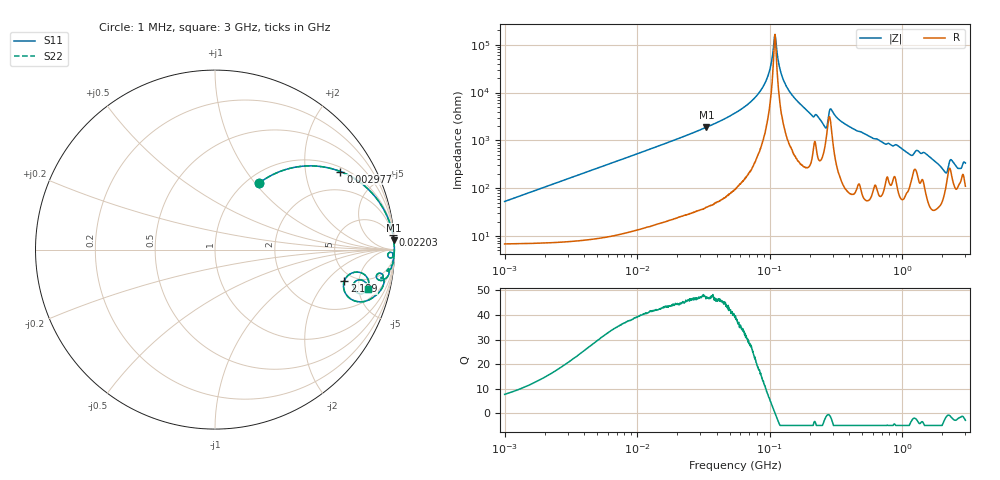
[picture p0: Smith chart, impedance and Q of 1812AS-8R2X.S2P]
!s-Parameter Generated by FASTRON Sdn. Bhd.
!FASTRON P/N : 1812AS-8R2X
!Keysight Technologies,E4991B,MY54100416,A.01.15
!Date created: Fri Oct 13 16:11:52 2023
!Version  : Rev00 Fri Oct 13 16:11:52 2023
!Data & Calibration Information:
!Freq	S11	S21	S12	S22
!PortZ  Port1:50+j0  Port2:50+j0
!When reading, reference impedance value at option line is always used.
! Remarks : This data is being provided solely for informational purposes.
# Hz S dB R 50
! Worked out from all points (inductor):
!   1601 points, 1 MHz to 3 GHz, reference 50 ohm
!   read as one part in series: L = 8.32 uH near 1.041 MHz
!   highest Q = 47.4 at 33.37 MHz (marker M1), where L = 8.97 uH
!   self-resonance near 109.3 MHz
!   S11 on the Smith chart (normalised r, x): 1 MHz: 1.14, +1.05; 2.977 MHz: 1.15, +3.11; 22.03 MHz: 2, +24; 2.189 GHz: 4.16, -3.22; 3 GHz: 3.20, -6.35
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1000000  -7.06 56.5  -1.51 -26.1  -1.51 -26.1  -7.06 56.5
2976856  -1.69 31.9  -5.53 -55.3  -5.53 -55.3  -1.69 31.9
3804036  -1.12 26.2  -7.08 -61.4  -7.08 -61.4  -1.12 26.2
1.447069e7  -0.10 7.5  -17.73 -81.2  -17.73 -81.2  -0.10 7.5
2.20312e7  -0.05 4.8  -21.48 -83.9  -21.48 -83.9  -0.05 4.8
3.337442e7  -0.02 3.0  -25.51 -85.7  -25.51 -85.7  -0.02 3.0
5.477226e7  -0.01 1.5  -31.39 -87.0  -31.39 -87.0  -0.01 1.5
8.854986e7  -0.01 0.4  -42.14 -85.3  -42.14 -85.3  -0.01 0.4
9.885493e7  -0.01 0.2  -48.34 -80.8  -48.34 -80.8  -0.01 0.2
1.098084e8  -0.01 -0.0  -64.28 3.6  -64.28 3.6  -0.01 -0.0
1.213667e8  -0.01 -0.2  -48.46 80.4  -48.46 80.4  -0.01 -0.2
1.328058e8  -0.01 -0.4  -42.93 84.1  -42.93 84.1  -0.01 -0.4
2.083556e8  -0.04 -1.7  -30.44 81.3  -30.44 81.3  -0.04 -1.7
2.622844e8  -0.20 -2.7  -25.62 62.3  -25.62 62.3  -0.20 -2.7
2.92808e8  -0.08 -1.2  -32.88 66.3  -32.88 66.3  -0.08 -1.2
4.033367e8  -0.03 -3.0  -25.65 84.7  -25.65 84.7  -0.03 -3.0
7.925923e8  -0.21 -6.4  -18.93 74.5  -18.93 74.5  -0.21 -6.4
1.637435e9  -0.39 -12.6  -13.16 72.3  -13.16 72.3  -0.39 -12.6
2.188818e9  -2.60 -13.6  -9.65 32.0  -9.65 32.0  -2.60 -13.6
2.335937e9  -1.28 -10.5  -13.21 46.2  -13.21 46.2  -1.28 -10.5
2.660507e9  -1.74 -16.5  -9.98 47.3  -9.98 47.3  -1.74 -16.5
3e9  -1.08 -14.4  -11.61 56.5  -11.61 56.5  -1.08 -14.4
